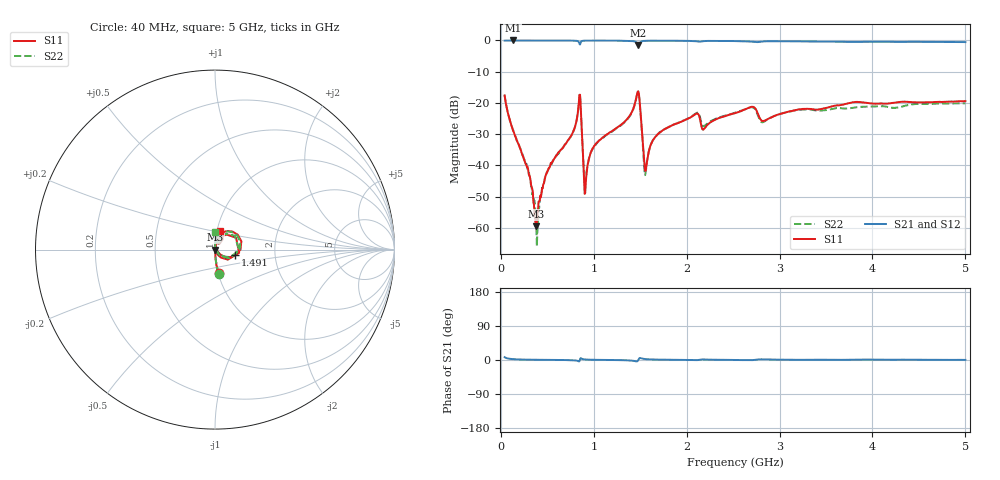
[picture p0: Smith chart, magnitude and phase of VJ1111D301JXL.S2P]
! VJ1111D301JXL
! DATE 02/15/2022  13:36
! CAPACITORS MOUNTED IN SERIES ON 25 MIL THICK MICROSTRIP SUBSTRATE
# GHz  S  MA  R  50.00
!  FREQ  S11M  S11A  S21M  S21A  S12M  S12A  S22M  S22A
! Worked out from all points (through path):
!   801 points, 40 MHz to 5 GHz, reference 50 ohm
!   highest |S21| = 0.00 dB at 126.8 MHz (marker M1); lowest = -1.4 dB at 1.478 GHz (marker M2)
!   lowest |S11| = -59.5 dB at 374.8 MHz (marker M3), VSWR 1.00, Z = 50.1 - j0.02 ohm
!   |S11| at or under -10 dB: start of sweep to end of sweep
!   |S22| runs from -65.8 to -16.5 dB; largest |S21 - S12| = 0.011
!   S11 on the Smith chart (normalised r, x): 40 MHz: 1.01, -0.27; 1.491 GHz: 1.25, -0.08; 5 GHz: 1.04, +0.22
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0.04  0.1314 -81.3  0.9916 7.5  0.9918 7.7  0.1352 -81.6
0.1268  0.03754 -87.4  0.9998 2.4  0.9987 2.4  0.03873 -85.6
0.2942  0.00846 -77.7  0.9974 0.9  1 0.8  0.008071 -82.9
0.3748  0.001058 -10.9  0.9961 0.6  1.001 0.6  0.00153 -48.4
0.4988  0.007878 82.7  0.9965 0.4  0.9999 0.5  0.007886 83.1
0.7654  0.03186 81.9  0.9929 -0.5  0.9977 -0.6  0.03138 86.3
0.8336  0.08318 63.4  0.9639 -3.0  0.9684 -3.0  0.08245 68.5
0.8708  0.03628 -59.7  0.9767 3.3  0.982 3.2  0.03647 -51.3
0.8894  0.009084 -58.0  0.9898 1.9  0.9938 2.0  0.01031 -42.6
0.9142  0.005476 62.5  0.9929 1.2  0.9981 1.2  0.006516 54.0
1.001  0.02031 86.1  0.9952 0.5  0.9981 0.4  0.01991 84.5
1.4784  0.154 17.4  0.8486 -0.1  0.8538 -0.2  0.1489 17.5
1.4908  0.1184 -15.6  0.8841 4.8  0.8897 4.8  0.1138 -15.6
1.559  0.008336 35.7  0.9876 2.3  0.9913 2.2  0.007819 48.9
1.6954  0.03217 86.6  0.9902 1.0  0.9952 0.9  0.03243 90.2
2.1046  0.06752 71.5  0.9697 -0.3  0.9738 -0.4  0.06922 78.0
2.52  0.06879 84.0  0.9779 0.1  0.9831 -0.0  0.06979 89.0
2.7122  0.0868 66.5  0.9486 -0.2  0.9536 -0.4  0.08489 71.2
2.8238  0.05152 68.0  0.9642 1.8  0.9695 1.7  0.04942 78.3
3.3508  0.07954 78.5  0.9596 0.6  0.9645 0.4  0.07759 88.6
4.1754  0.09832 75.2  0.9521 0.6  0.9597 0.4  0.08543 90.9
5  0.1071 73.5  0.9416 0.3  0.9473 0.1  0.09865 90.7
